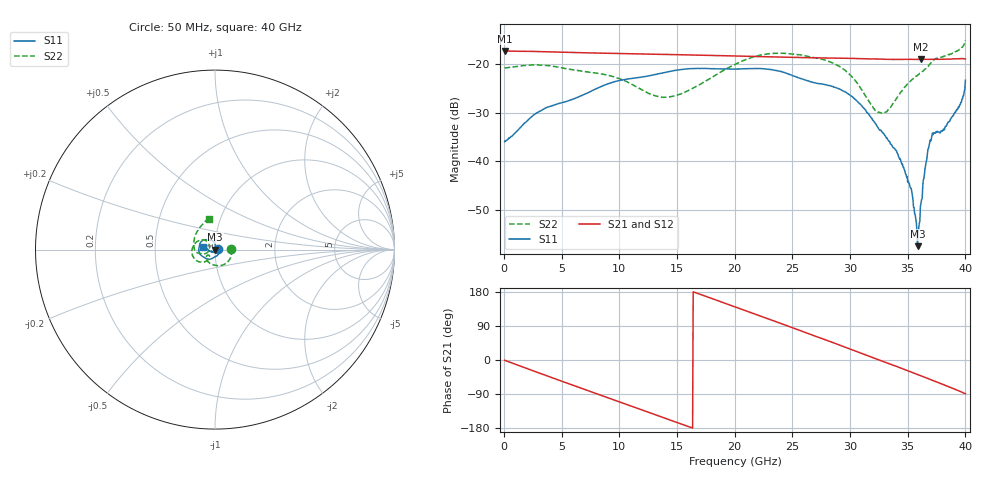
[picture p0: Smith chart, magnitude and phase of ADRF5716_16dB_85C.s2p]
! Device: ADRF5716
! Description: 30GHz 2-Bit Digital Attenuator
! Frequency: 100 MHz – 30 GHz
! Ports:
! ATTIN  = Port 1
! ATTOUT = Port 2
! State: 16 dB Attenuation selected
! Supply Voltage:
! VDD  =  +3.30 Volts
! VSS  =  -3.30 Volts
! Control Voltages:
! D5 = 3.3V, D6 = 0V
! Temperature = +85 C
! Data: Data was collected using a calibrated network analyzer.
!  The reference plane is the package pins of ADRF5716 switch.
! Note: Analog Devices supplies this data as a sample of measured data for this product.
!  Your particular data for this product may vary.
!  Analog Devices reserves the right to change this data at anytime
# HZ S DB R 50
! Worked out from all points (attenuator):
!   800 points, 50 MHz to 40 GHz, reference 50 ohm
!   highest |S21| = -17.25 dB at 100 MHz (marker M1); lowest = -19.0 dB at 36.15 GHz (marker M2)
!   lowest |S11| = -57.6 dB at 35.85 GHz (marker M3), VSWR 1.00, Z = 50.1 + j0.0465 ohm
!   |S11| at or under -10 dB: start of sweep to end of sweep
!   |S22| runs from -30.1 to -15.1 dB; largest |S21 - S12| = 0
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5e7  -36.00 5.9  -17.25 -0.6  -17.25 -0.6  -20.77 1.0
1e8  -35.76 0.7  -17.25 -1.2  -17.25 -1.2  -20.72 -0.8
2.85e9  -30.02 -53.4  -17.36 -32.1  -17.36 -32.1  -20.13 -42.9
6.75e9  -26.42 -102.9  -17.61 -75.0  -17.61 -75.0  -21.41 -97.4
9.7e9  -23.51 -127.6  -17.76 -107.2  -17.76 -107.2  -22.72 -129.2
1.34e10  -21.94 -152.1  -17.93 -147.5  -17.93 -147.5  -26.68 -139.6
1.545e10  -21.06 -165.4  -18.03 -169.8  -18.03 -169.8  -26.03 -127.6
2.005e10  -20.97 168.0  -18.28 139.8  -18.28 139.8  -19.97 -135.4
2.315e10  -21.08 147.9  -18.46 105.9  -18.46 105.9  -17.77 -163.2
2.67e10  -23.67 127.5  -18.65 66.2  -18.65 66.2  -18.54 166.4
3.01e10  -26.58 100.6  -18.77 27.8  -18.77 27.8  -22.40 137.2
3.225e10  -32.37 85.4  -18.91 3.1  -18.91 3.1  -29.70 154.4
3.335e10  -35.84 86.0  -18.99 -9.4  -18.99 -9.4  -29.37 -171.8
3.42e10  -39.05 83.3  -18.99 -18.9  -18.99 -18.9  -26.43 -158.2
3.515e10  -44.74 81.5  -18.97 -29.9  -18.97 -29.9  -23.65 -159.0
3.585e10  -57.57 20.5  -18.98 -38.1  -18.98 -38.1  -22.27 -162.8
3.6e10  -52.91 -30.0  -18.98 -39.9  -18.98 -39.9  -21.98 -163.5
3.615e10  -48.59 -61.8  -19.00 -41.7  -19.00 -41.7  -21.75 -164.7
3.655e10  -40.83 -90.3  -18.97 -46.4  -18.97 -46.4  -20.92 -166.8
3.705e10  -35.41 -118.4  -18.97 -52.5  -18.97 -52.5  -19.58 -172.0
3.935e10  -29.22 -172.4  -18.86 -80.4  -18.86 -80.4  -17.18 138.4
4e10  -23.30 167.3  -18.91 -89.1  -18.91 -89.1  -15.07 101.5
